| IBIS file stm32u073_083_ufqfpn32.ibs
[IBIS ver] 4.2
[File name] stm32u073_083_ufqfpn32.ibs
[File Rev] 0.3
[Date] 20-02-2024
[Source] Data Created at STMicroelectronics
[Notes]  File originated from ELDO simulations.
[Disclaimer]  This information is for modeling purpose only and is
   not guaranteed. The information is subject to change without
   notice.
[Copyright] Copyright 2024 STMicroelectronics Inc.
|   Component stm32u073_083_ufqfpn32
[Component] stm32u073_083_ufqfpn32
[Manufacturer] STMicroelectronics
[Package]
| variable   typ   min   max
R_pkg  0  NA  NA
L_pkg  0  NA  NA
C_pkg  0  NA  NA
[Pin]   signal_name   model_name
1  VDD  power
2  PC14-OSC32_IN  io8_ft_v33
3  PC15-OSC32_OUT  io8_ft
4  PF2-NRST  ioreset_ft_v33
5  VDDA_VREFP  nc
6  PA0-CK_IN  io8_ft_v33
7  PA1  io8_ft_v33
8  PA2  io8_ft_v33
9  PA3  io8_ft
10  PA4  io8_ft
11  PA5  io8_ft
12  PA6  io8_ft_i2c
13  PA7  io8_ft_i2c
14  PB0  io8_ft
15  PB1  io8_ft
16  VSS  gnd
17  VDDUSB  power
18  PA8  io8_ft
19  PA9  io8_ft_i2c
20  PA10  io8_ft_i2c
21  PA11  io8usb_ft_phy
22  PA12  io8usb_ft_phy
23  PA13  io8_ft
24  PA14  io8_ft
25  PA15  io8_ft
26  PB3  io8_ft_i2c
27  PB4  io8_ft_i2c
28  PB5  io8_ft
29  PB6  io8_ft_i2c
30  PB7  io8_ft_i2c
31  PF3-BOOT0  io8_ft_v33
32  VSS  gnd
[Package Model]   489-qfpn-5x5-32-ldo-240125
[Pin Mapping]   pulldown_ref   pullup_ref   | Comment
1  nc  vddio
2  gndio  vddio  | Depending on IO usage
| 2  gndio   | Depending on IO usage
3  gndio  vddio  | Depending on IO usage
| 3  gndio   | Depending on IO usage
4  gndio  vddio
5  nc  nc
6  gndio  vddio
7  gndio  vddio
8  gndio  vddio
9  gndio  vddio
10  gndio  vddio
11  gndio  vddio
12  gndio  vddio
13  gndio  vddio
14  gndio  vddio
15  gndio  vddio
16  gndio  nc
17  nc  vddio
18  gndio  vddio
19  gndio  vddio
20  gndio  vddio
21  gndio  vddio
22  gndio  vddio
23  gndio  vddio
24  gndio  vddio
25  gndio  vddio
26  gndio  vddio
27  gndio  vddio
28  gndio  vddio
29  gndio  vddio
30  gndio  vddio
31  gndio  vddio
32  gndio  nc
|[Diff Pin]  inv_pin  vdiff  tdelay_typ  tdelay_min  tdelay_max
|22  21  NA  NA  NA  NA
[Model Selector] io8_ft
io8_ft_ls_1v2   "GPIO - 5V tolerant - 1.2V range - Low speed"
io8_ft_ms_1v2   "GPIO - 5V tolerant - 1.2V range - Med speed"
io8_ft_fs_1v2   "GPIO - 5V tolerant - 1.2V range - Fast speed"
io8_ft_hs_1v2   "GPIO - 5V tolerant - 1.2V range - High speed"
io8_ft_ls_1v8   "GPIO - 5V tolerant - 1.8V range - Low speed"
io8_ft_ms_1v8   "GPIO - 5V tolerant - 1.8V range - Med speed"
io8_ft_fs_1v8   "GPIO - 5V tolerant - 1.8V range - Fast speed"
io8_ft_hs_1v8   "GPIO - 5V tolerant - 1.8V range - High speed"
io8_ft_ls_3v3   "GPIO - 5V tolerant - 3.3V range - Low speed"
io8_ft_ms_3v3   "GPIO - 5V tolerant - 3.3V range - Med speed"
io8_ft_fs_3v3   "GPIO - 5V tolerant - 3.3V range - Fast speed"
io8_ft_hs_3v3   "GPIO - 5V tolerant - 3.3V range - High speed"
[Model Selector] io8_ft_i2c
io8_ft_ls_1v2   "GPIO - 5V tolerant - 1.2V range - Low speed"
io8_ft_ms_1v2   "GPIO - 5V tolerant - 1.2V range - Med speed"
io8_ft_fs_1v2   "GPIO - 5V tolerant - 1.2V range - Fast speed"
io8_ft_hs_1v2   "GPIO - 5V tolerant - 1.2V range - High speed"
io8_ft_ls_1v8   "GPIO - 5V tolerant - 1.8V range - Low speed"
io8_ft_ms_1v8   "GPIO - 5V tolerant - 1.8V range - Med speed"
io8_ft_fs_1v8   "GPIO - 5V tolerant - 1.8V range - Fast speed"
io8_ft_hs_1v8   "GPIO - 5V tolerant - 1.8V range - High speed"
io8_ft_ls_3v3   "GPIO - 5V tolerant - 3.3V range - Low speed"
io8_ft_ms_3v3   "GPIO - 5V tolerant - 3.3V range - Med speed"
io8_ft_fs_3v3   "GPIO - 5V tolerant - 3.3V range - Fast speed"
io8_ft_hs_3v3   "GPIO - 5V tolerant - 3.3V range - High speed"
io8_ft_i2c_ls_1v2   "GPIO I2C open-drain - 5V tolerant - 1.2V range - Low speed"
io8_ft_i2c_ms_1v2   "GPIO I2C open-drain - 5V tolerant - 1.2V range - Med speed"
io8_ft_i2c_fs_1v2   "GPIO I2C open-drain - 5V tolerant - 1.2V range - Fast speed"
io8_ft_i2c_hs_1v2   "GPIO I2C open-drain - 5V tolerant - 1.2V range - High speed"
io8_ft_i2c_ls_1v8   "GPIO I2C open-drain - 5V tolerant - 1.8V range - Low speed"
io8_ft_i2c_ms_1v8   "GPIO I2C open-drain - 5V tolerant - 1.8V range - Med speed"
io8_ft_i2c_fs_1v8   "GPIO I2C open-drain - 5V tolerant - 1.8V range - Fast speed"
io8_ft_i2c_hs_1v8   "GPIO I2C open-drain - 5V tolerant - 1.8V range - High speed"
io8_ft_i2c_ls_3v3   "GPIO I2C open-drain - 5V tolerant - 3.3V range - Low speed"
io8_ft_i2c_ms_3v3   "GPIO I2C open-drain - 5V tolerant - 3.3V range - Med speed"
io8_ft_i2c_fs_3v3   "GPIO I2C open-drain - 5V tolerant - 3.3V range - Fast speed"
io8_ft_i2c_hs_3v3   "GPIO I2C open-drain - 5V tolerant - 3.3V range - High speed"
io8_ft_i2c_fmp_3v3   "GPIO I2C open-drain fm+ - 5V tolerant - 3.3V range"
[Model Selector] io8_ft_v33
io8_ft_v33_ls_1v2   "GPIO_V33 - 5V tolerant - 1.2V range - Low speed"
io8_ft_v33_ms_1v2   "GPIO_V33 - 5V tolerant - 1.2V range - Med speed"
io8_ft_v33_fs_1v2   "GPIO_V33 - 5V tolerant - 1.2V range - Fast speed"
io8_ft_v33_hs_1v2   "GPIO_V33 - 5V tolerant - 1.2V range - High speed"
io8_ft_v33_ls_1v8   "GPIO_V33 - 5V tolerant - 1.8V range - Low speed"
io8_ft_v33_ms_1v8   "GPIO_V33 - 5V tolerant - 1.8V range - Med speed"
io8_ft_v33_fs_1v8   "GPIO_V33 - 5V tolerant - 1.8V range - Fast speed"
io8_ft_v33_hs_1v8   "GPIO_V33 - 5V tolerant - 1.8V range - High speed"
io8_ft_v33_ls_3v3   "GPIO_V33 - 5V tolerant - 3.3V range - Low speed"
io8_ft_v33_ms_3v3   "GPIO_V33 - 5V tolerant - 3.3V range - Med speed"
io8_ft_v33_fs_3v3   "GPIO_V33 - 5V tolerant - 3.3V range - Fast speed"
io8_ft_v33_hs_3v3   "GPIO_V33 - 5V tolerant - 3.3V range - High speed"
[Model Selector] io8usb_ft_phy
io8_ft_ls_1v2   "GPIO - 5V tolerant - 1.2V range - Low speed"
io8_ft_ms_1v2   "GPIO - 5V tolerant - 1.2V range - Med speed"
io8_ft_fs_1v2   "GPIO - 5V tolerant - 1.2V range - Fast speed"
io8_ft_hs_1v2   "GPIO - 5V tolerant - 1.2V range - High speed"
io8_ft_ls_1v8   "GPIO - 5V tolerant - 1.8V range - Low speed"
io8_ft_ms_1v8   "GPIO - 5V tolerant - 1.8V range - Med speed"
io8_ft_fs_1v8   "GPIO - 5V tolerant - 1.8V range - Fast speed"
io8_ft_hs_1v8   "GPIO - 5V tolerant - 1.8V range - High speed"
io8_ft_ls_3v3   "GPIO - 5V tolerant - 3.3V range - Low speed"
io8_ft_ms_3v3   "GPIO - 5V tolerant - 3.3V range - Med speed"
io8_ft_fs_3v3   "GPIO - 5V tolerant - 3.3V range - Fast speed"
io8_ft_hs_3v3   "GPIO - 5V tolerant - 3.3V range - High speed"
io8usb_ft_phy_hs_3v3   "USB full speed"
io8usb_ft_phy_ls_3v3   "USB low speed"
[Model Selector] ioreset_ft_v33
ioreset_ft_v33_1v2   "Reset PAD. 5V tolerant. 1.2V range"
ioreset_ft_v33_1v8   "Reset PAD. 5V tolerant. 1.8V range"
ioreset_ft_v33_3v3   "Reset PAD. 5V tolerant. 3.3V range"
[Define Package Model]  489-qfpn-5x5-32-ldo-240125
[Manufacturer]  Unknown
[OEM]  Unknown
[Description]  None
[Number Of Pins]  32
[Pin Numbers]
| Pin Num   Terminal Name
6 | PA0-CK_IN
20 | PA10
21 | PA11
22 | PA12
23 | PA13
24 | PA14
25 | PA15
7 | PA1
8 | PA2
9 | PA3
10 | PA4
11 | PA5
12 | PA6
13 | PA7
18 | PA8
19 | PA9
14 | PB0
15 | PB1
26 | PB3
27 | PB4
28 | PB5
29 | PB6
30 | PB7
2 | PC14-OSC32_IN
3 | PC15-OSC32_OUT
4 | PF2-NRST
31 | PF3-BOOT0
1 | VDD
17 | VDDUSB
5 | VDDA_VREFP
16 | VSS
32 | VSS
[Model Data]
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[End Model Data]
[End Package Model]
|End [Component]
| Models and submodels in the file (42): io8_ft_fs_1v2 (I/O), io8_ft_fs_1v8 (I/O), io8_ft_fs_3v3 (I/O), io8_ft_hs_1v2 (I/O), io8_ft_hs_1v8 (I/O), io8_ft_hs_3v3 (I/O), io8_ft_i2c_fmp_3v3 (I/O_open_drain), io8_ft_i2c_fs_1v2 (I/O_open_drain), io8_ft_i2c_fs_1v8 (I/O_open_drain), io8_ft_i2c_fs_3v3 (I/O_open_drain), io8_ft_i2c_hs_1v2 (I/O_open_drain), io8_ft_i2c_hs_1v8 (I/O_open_drain), io8_ft_i2c_hs_3v3 (I/O_open_drain), io8_ft_i2c_ls_1v2 (I/O_open_drain), io8_ft_i2c_ls_1v8 (I/O_open_drain), io8_ft_i2c_ls_3v3 (I/O_open_drain), io8_ft_i2c_ms_1v2 (I/O_open_drain), io8_ft_i2c_ms_1v8 (I/O_open_drain), io8_ft_i2c_ms_3v3 (I/O_open_drain), io8_ft_ls_1v2 (I/O), io8_ft_ls_1v8 (I/O), io8_ft_ls_3v3 (I/O), io8_ft_ms_1v2 (I/O), io8_ft_ms_1v8 (I/O), io8_ft_ms_3v3 (I/O), io8_ft_v33_fs_1v2 (I/O), io8_ft_v33_fs_1v8 (I/O), io8_ft_v33_fs_3v3 (I/O), io8_ft_v33_hs_1v2 (I/O), io8_ft_v33_hs_1v8 (I/O), io8_ft_v33_hs_3v3 (I/O), io8_ft_v33_ls_1v2 (I/O), io8_ft_v33_ls_1v8 (I/O), io8_ft_v33_ls_3v3 (I/O), io8_ft_v33_ms_1v2 (I/O), io8_ft_v33_ms_1v8 (I/O), io8_ft_v33_ms_3v3 (I/O), io8usb_ft_phy_hs_3v3 (I/O), io8usb_ft_phy_ls_3v3 (I/O), ioreset_ft_v33_1v2 (I/O_open_drain), ioreset_ft_v33_1v8 (I/O_open_drain), ioreset_ft_v33_3v3 (I/O_open_drain)
